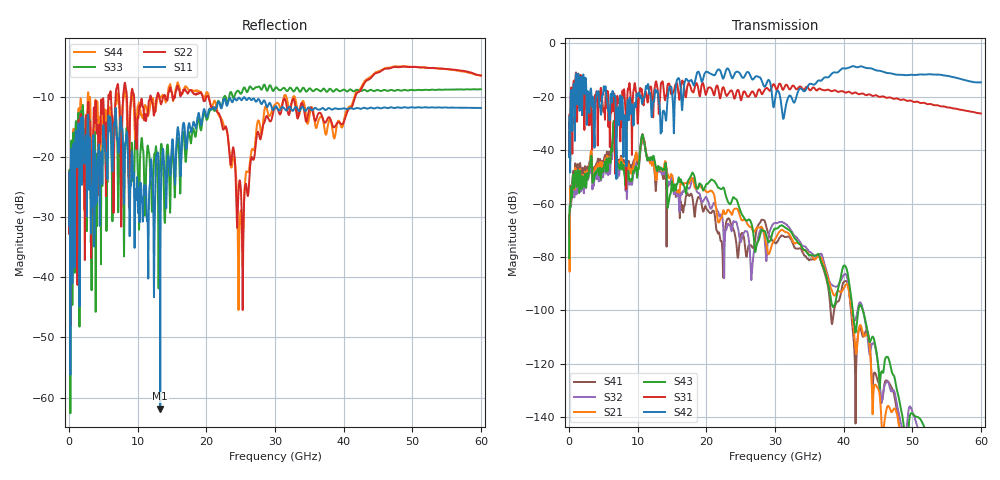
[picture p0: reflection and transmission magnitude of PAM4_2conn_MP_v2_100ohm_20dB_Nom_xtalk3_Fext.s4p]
! Info: Touchstone file created by Circ.  Input file=FAB50GbE_2conn_Midplane_Examax_Topo2_v2_100ohm_20dB_Nom.circ
# Hz S RI R 50
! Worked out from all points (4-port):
!   6000 points, 10 MHz to 60 GHz, reference 50 ohm
!   strongest paths, dB at 10 MHz, 15.01 GHz, 30.01 GHz, 45.01 GHz, 60 GHz:
!     S42: -42.6, -18.4, -20.8, -10.2, -14.6
!     S31: -41.9, -18.9, -16.0, -19.8, -26.2
!     S43: -80.4, -51.6, -69.3, -119.9, -160.3
!     S21: -64.1, -49.3, -73.2, -129.2, -166.1
!     S32: -68.2, -50.1, -67.2, -119.8, -164.2
!     S41: -67.5, -50.8, -74.7, -126.6, -179.5
!   lowest |S11| = -61.9 dB at 13.28 GHz (marker M1), VSWR 1.00, Z = 50.1 - j0.0479 ohm
!   |S11| at or under -10 dB: start of sweep to 25.45 GHz; 25.57 GHz to end of sweep
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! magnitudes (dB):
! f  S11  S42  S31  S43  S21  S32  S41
! 10 MHz  -31.4  -42.6  -41.9  -80.4  -64.1  -68.2  -67.5
! 1.2 GHz  -21.3  -21.6  -21.3  -49.7  -48.5  -50.6  -46.3
! 6.41 GHz  -18.6  -18.9  -22.6  -31.5  -34.7  -36.4  -32.3
! 13.28 GHz  -61.9  -28.2  -18.9  -46.6  -46.7  -47.9  -46.9
! 24.87 GHz  -10.2  -11.1  -19.4  -62.0  -64.4  -73.6  -73.8
! 28.66 GHz  -11.1  -15.7  -16.9  -71.4  -74.4  -79.0  -67.9
! 60 GHz  -11.8  -14.6  -26.2  -160.3  -166.1  -164.2  -179.5
